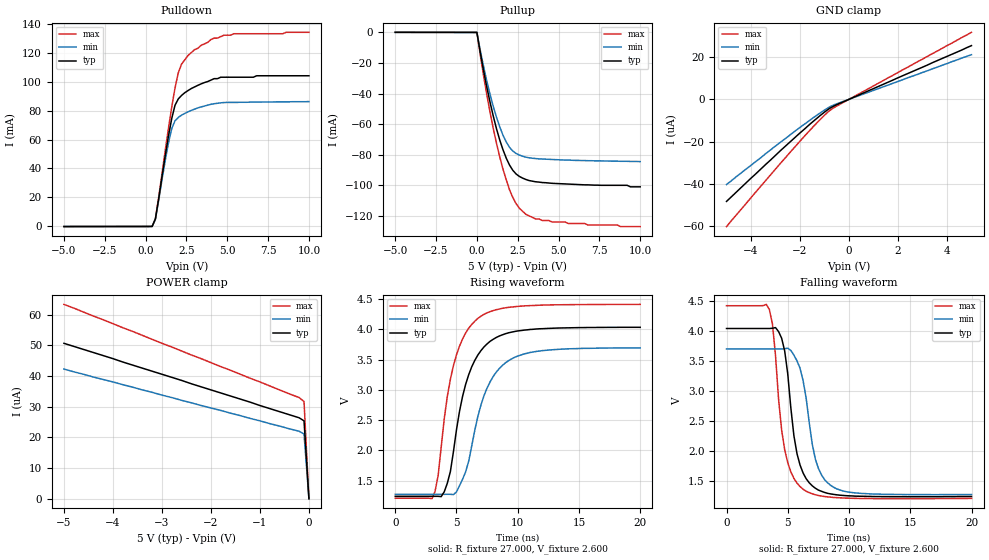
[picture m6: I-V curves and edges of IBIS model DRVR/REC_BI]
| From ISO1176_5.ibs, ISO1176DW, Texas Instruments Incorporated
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|   Driver Output / Receiver Input Model
[Model]   DRVR/REC_BI
Model_type   I/O
| Signals   A,B
Vinl = 0.9V
Vinh = 2.8V
Vmeas = 1.7V   |Reference voltage for timing measurements
Cref = 50pF   |Timing specification test load capacitance value
Rref = 54   |Note: 54 Ohm load; single-ended configuration
|   Timing specification test load voltage
| variable   typ   min   max
C_comp   7pF   5.6pF   8.4pF
|   typ   min   max
[Temperature Range]   25.0   -40   85
[Voltage range]   5.0V   4.5V   5.5V
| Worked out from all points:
|   slope of the pulldown table from 0 to 0.75 V, typ, clamps not added: 48.2 ohm
|   slope of the pullup table from 0 to 0.75 V, typ, clamps not added: 17.5 ohm
|   rising waveform, R_fixture 27.000, V_fixture 2.600: 20-80 % time 1.85ns typ, 2.06ns min, 1.71ns max; typ from 1.24 V to 4.04 V
|   falling waveform, R_fixture 27.000, V_fixture 2.600: 20-80 % time 1.09ns typ, 1.22ns min, 1.03ns max; typ from 4.04 V to 1.24 V
[Pulldown]
|   Voltage   I(typ)   I(min)   I(max)
-5V       -76.3uA    -63.7uA    -95.2uA
400mV     11.4uA     14.8uA     6.13uA
600mV     5.13mA     4.94mA     5.34mA
1.4V      62.4mA     57.6mA     67.8mA
1.6V      74.5mA     67.5mA     82.4mA
1.8V      83.6mA     72.9mA     95.5mA
2V        88mA       75.2mA     106mA
2.2V      90.4mA     76.8mA     112mA
3V        96.3mA     81mA       122mA
4V        101mA      84.3mA     129mA
4.8V      103mA      85.5mA     132mA
10V       104mA      86.2mA     134mA
[Pullup]
|   Voltage   I(typ)   I(min)   I(max)
| Note that the[Pullup]voltage table is referenced to Vcc
| and is calculated using Vtable=Vcc - Vmeasured.
-5V       83.5uA     69.6uA     105uA
0V        18.8uA     16.3uA     22.1uA
400mV     -24.4mA    -21.8mA    -27.7mA
800mV     -45.4mA    -40.3mA    -51.9mA
1.2V      -63mA      -55.5mA    -72.5mA
1.6V      -76.8mA    -67.3mA    -89.5mA
2V        -86.8mA    -75.2mA    -103mA
2.2V      -90.2mA    -77.6mA    -108mA
2.6V      -94.2mA    -80.2mA    -115mA
3V        -96.2mA    -81.6mA    -119mA
4.6V      -98.7mA    -83.1mA    -124mA
10V       -101mA     -84.5mA    -127mA
[GND_clamp]
|   Voltage  I(typ)   I(min)   I(max)
| Outputs in High Impedance (off)
-5V       -48.3uA    -40.3uA    -60.2uA
-2.4V     -20.1uA    -16.8uA    -25uA
-1.4V     -9.84uA    -8.24uA    -12.2uA
-800mV    -4.35uA    -3.65uA    -5.4uA
-400mV    -2.03uA    -1.69uA    -2.54uA
5V        25.4uA     21.1uA     31.7uA
[POWER_clamp]
|   Voltage  I(typ)   I(min)   I(max)
| Note that the [POWER_clamp] voltage table is referenced to Vcc
| and is calculated using Vtable = Vcc - Vmeasured.
| Outputs in Tri-state.
-5V       50.7uA     42.3uA     63.4uA
-200mV    26.4uA     22uA       33uA
-100mV    25.4uA     21.1uA     31.7uA
0V        0A         0A         0A
[Ramp]
|   typ   min   max
dV/dt_r   2.30V/3.19ns   2.21V/3.52ns  2.38V/2.84ns
dV/dt_f   2.29V/1.94ns   2.20V/2.18ns  2.37V/1.80ns
R_load = 27ohm | Note: The measurement is on a single-ended configuration
|   with 54ohm line-to-line.
[Rising Waveform]
R_fixture = 27.000
V_fixture = 2.600
V_fixture_min = 2.600
V_fixture_max = 2.600
C_fixture = 0.000
L_fixture = 0.000
|  time   V(typ)   V(min)   V(max)
0s        1.24V      1.273V     1.208V
3ns       1.24V      1.273V     1.201V
3.5ns     1.24V      1.273V     1.58V
4ns       1.314V     1.273V     2.522V
4.75ns    1.977V     1.268V     3.401V
5.5ns     2.896V     1.523V     3.845V
6.75ns    3.579V     2.565V     4.184V
8ns       3.838V     3.223V     4.313V
9.75ns    3.967V     3.54V      4.377V
20ns      4.036V     3.696V     4.415V
[Falling Waveform]
R_fixture = 27.000
V_fixture = 2.600
V_fixture_min = 2.600
V_fixture_max = 2.600
C_fixture = 0.000
L_fixture = 0.000
|  time   V(typ)   V(min)   V(max)
0s        4.036V     3.696V     4.415V
3.5ns     4.036V     3.696V     4.35V
3.75ns    4.04V      3.696V     4.109V
4.25ns    3.984V     3.696V     2.858V
4.75ns    3.66V      3.699V     2.017V
5.5ns     2.253V     3.593V     1.542V
6.25ns    1.632V     3.171V     1.362V
7.25ns    1.378V     1.864V     1.269V
8.5ns     1.283V     1.426V     1.229V
20ns      1.24V      1.273V     1.208V
